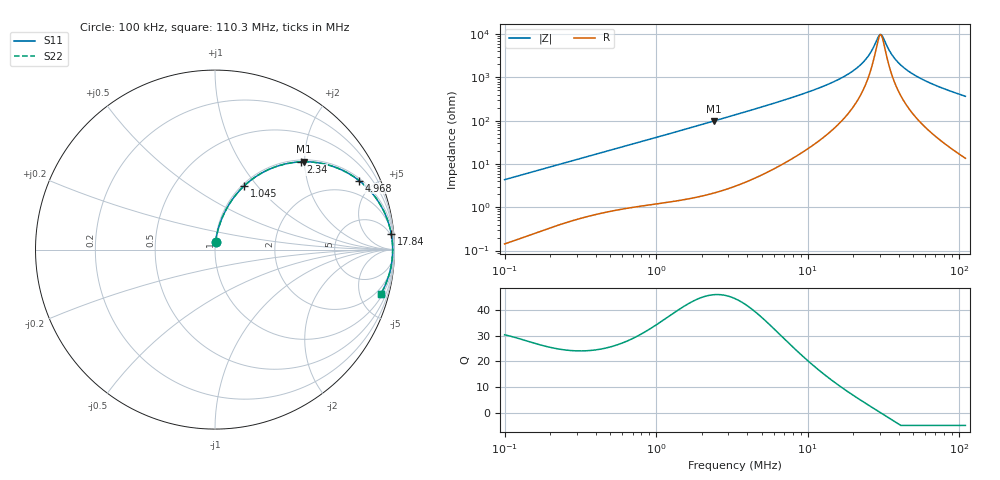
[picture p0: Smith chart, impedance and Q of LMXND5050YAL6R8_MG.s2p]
! LMXND5050YAL6R8_MG  S-PARAMETER MODEL  ( General Type )
! Model Generated by TAIYO YUDEN Corporation (https://www.yuden.co.jp/en/)
! Version 1.0
! TAIYO YUDEN Control No. 191023NI43SB-FBB
! Copyright(c) 2019 TAIYO YUDEN CO.,LTD. All Rights Reserved.
! Product Description (link to TY-COMPAS)
! https://ds.yuden.co.jp/TYCOMPAS/or/detail?pn=LMXND5050YAL6R8MMG&u=M
! Products Name : Inductors
! Characteristics :
!  Inductance : 6.8 uH , SRF(min) : 21 MHz , DC Resistance(max) : 0.0637 Ohm
!  Rated Current : Saturation :2800 mA , Temp Rise : 2400 mA (40 degC)
!  Case Size : 4.9 x 4.9 / 0.193 x 0.193 [mm/inch] , Thickness : 4.1 / 0.161 [mm/inch]
!  (Conditions: Temperature = 25 degC , DC Bias Current/Voltage = 0A / 0V)
! External Node Assignments :
!  1  o---GGG---o  2
! GND o---------o GND
! Frequency Range : 0.1MHz  -  110.285862MHz  [ 402 STEP ]
# MHz S RI R 50
! Freq[MHz].  S11 Real  S11 Imag  S21 Real  S21 Imag  S12 Real  S12 Imag  S22 Real  S22 Imag
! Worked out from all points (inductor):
!   401 points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, 100 kHz to 110.3 MHz, reference 50 ohm
!   read as one part in series: L = 6.87 uH near 103.6 kHz
!   highest Q = 46.1 at 2.423 MHz (marker M1), where L = 6.49 uH
!   self-resonance near 30.18 MHz
!   S11 on the Smith chart (normalised r, x): 100 kHz: 1.00, +0.09; 1.045 MHz: 1.02, +0.85; 2.34 MHz: 1.04, +1.91; 4.968 MHz: 1.11, +4.13; 17.84 MHz: 3, +22; 110.3 MHz: 1.27, -7.30
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0.1  0.00329 0.0431  0.9967 -0.0431  0.9967 -0.0431  0.00329 0.0431
0.323312  0.0235 0.1321  0.9765 -0.1321  0.9765 -0.1321  0.0235 0.1321
0.629016  0.0706 0.2387  0.9294 -0.2387  0.9294 -0.2387  0.0706 0.2387
1.045308  0.1611 0.3536  0.8389 -0.3536  0.8389 -0.3536  0.1611 0.3536
1.509998  0.2791 0.4366  0.7209 -0.4366  0.7209 -0.4366  0.2791 0.4366
2.339559  0.4767 0.4887  0.5233 -0.4887  0.5233 -0.4887  0.4767 0.4887
2.422962  0.4939 0.4892  0.5061 -0.4892  0.5061 -0.4892  0.4939 0.4892
3.320932  0.646 0.4671  0.354 -0.4671  0.354 -0.4671  0.646 0.4671
4.968266  0.8036 0.3841  0.1964 -0.3841  0.1964 -0.3841  0.8036 0.3841
10.73698  0.9516 0.1897  0.0484 -0.1897  0.0484 -0.1897  0.9516 0.1897
17.84287  0.9819 0.0882  0.0181 -0.0882  0.0181 -0.0882  0.9819 0.0882
21.25826  0.9865 0.0579  0.0135 -0.0579  0.0135 -0.0579  0.9865 0.0579
24.031  0.9885 0.0376  0.0115 -0.0376  0.0115 -0.0376  0.9885 0.0376
26.2303  0.9893 0.0234  0.0107 -0.0234  0.0107 -0.0234  0.9893 0.0234
29.13675  0.9899 0.00657  0.0101 -0.00657  0.0101 -0.00657  0.9899 0.00657
30.17544  0.9899 0.000976  0.0101 -0.000976  0.0101 -0.000976  0.9899 0.000976
31.25117  0.9899 -0.00462  0.0101 0.00462  0.0101 0.00462  0.9899 -0.00462
34.71395  0.9895 -0.0214  0.0105 0.0214  0.0105 0.0214  0.9895 -0.0214
40.64066  0.9877 -0.0471  0.0123 0.0471  0.0123 0.0471  0.9877 -0.0471
51.03201  0.9824 -0.086  0.0176 0.086  0.0176 0.086  0.9824 -0.086
71.18072  0.9668 -0.1495  0.0332 0.1495  0.0332 0.1495  0.9668 -0.1495
110.2859  0.9224 -0.2497  0.0776 0.2497  0.0776 0.2497  0.9224 -0.2497
